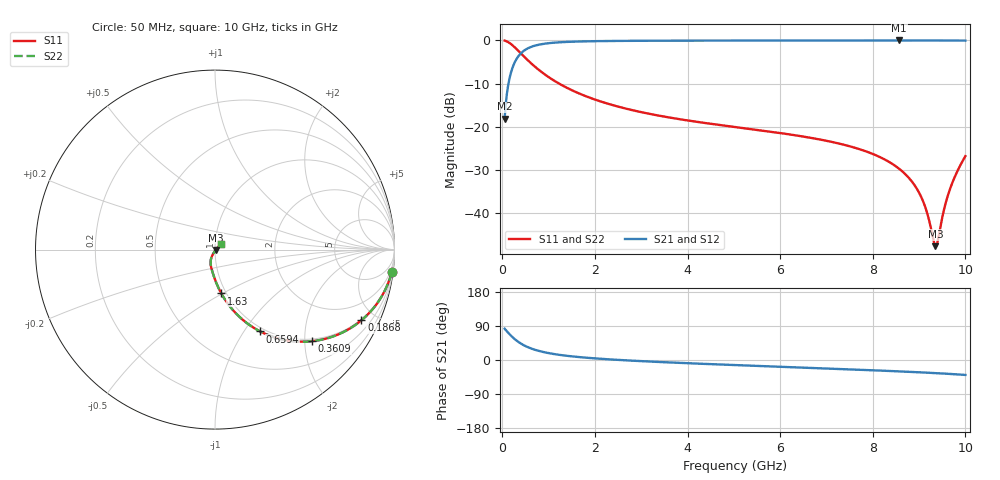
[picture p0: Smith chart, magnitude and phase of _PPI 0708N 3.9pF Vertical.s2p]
! S-Parameter data specifications (vertical orientation):
! Substrate: 40-mil Rogers 3003C, Substrate thickness, H=1.016mm, Dielectric constant, Er=3, Conductor thickness, T_mtl=0.043mm, Loss Tangent, Tand=0.003
! PCB Mounting Pad Footprint: Pad width, PadW=2.54mm , Pad length, PadL=0.51mm , Pad gap, PadG (edge-to-edge)=0.71mm , Reference planes=1.73mm apart
! Created Tue Jan 16 08:45:19 2018
# GHz S MA R 50
! 2 Port Network Data from SP1.SP block
! freq  magS11  angS11  magS21  angS21  magS12  angS12  magS22  angS22
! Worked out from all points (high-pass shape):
!   801 points, 50 MHz to 10 GHz, reference 50 ohm
!   highest |S21| = -0.03 dB at 8.57 GHz (marker M1); lowest = -18.1 dB at 50 MHz (marker M2)
!   |S21| within 3 dB of the highest: 399 MHz to end of sweep
!   lowest |S11| = -47.6 dB at 9.353 GHz (marker M3), VSWR 1.01, Z = 50.3 - j0.279 ohm
!   |S11| at or under -10 dB: 1.226 GHz to end of sweep
!   |S22| runs from -47.6 to -0.1 dB; largest |S21 - S12| = 0
!   S11 on the Smith chart (normalised r, x): 50 MHz: 1, -16; 186.8 MHz: 0.95, -4.17; 360.9 MHz: 0.95, -2.16; 659.4 MHz: 0.95, -1.19; 1.63 GHz: 0.95, -0.49; 10 GHz: 1.07, +0.07
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0.05  0.9923 -7.3  0.1241 82.7  0.1241 82.7  0.9923 -7.3
0.1370625  0.9459 -19.4  0.3241 70.5  0.3241 70.5  0.9459 -19.4
0.1868125  0.906 -25.7  0.423 64.2  0.423 64.2  0.906 -25.7
0.3609375  0.7428 -43.4  0.6691 46.6  0.6691 46.6  0.7428 -43.4
0.6594375  0.5208 -61.1  0.8531 28.8  0.8531 28.8  0.5208 -61.1
1.032563  0.366 -72.4  0.9299 17.5  0.9299 17.5  0.366 -72.4
1.629563  0.2471 -81.8  0.9681 8.0  0.9681 8.0  0.2471 -81.8
1.716625  0.2362 -82.8  0.9708 7.1  0.9708 7.1  0.2362 -82.8
3.370812  0.1352 -94.7  0.9895 -5.1  0.9895 -5.1  0.1352 -94.7
5.025  0.09969 -102.6  0.9933 -13.4  0.9933 -13.4  0.09969 -102.6
6.691625  0.07427 -109.5  0.9951 -21.0  0.9951 -21.0  0.07427 -109.5
7.674188  0.05615 -113.2  0.9958 -25.5  0.9958 -25.5  0.05615 -113.2
8.345812  0.03959 -114.9  0.9961 -28.8  0.9961 -28.8  0.03959 -114.9
8.569688  0.03284 -114.8  0.9962 -30.0  0.9962 -30.0  0.03284 -114.8
8.830875  0.02389 -113.6  0.9961 -31.4  0.9961 -31.4  0.02389 -113.6
9.029875  0.01617 -109.9  0.996 -32.6  0.996 -32.6  0.01617 -109.9
9.15425  0.01097 -103.3  0.9958 -33.3  0.9958 -33.3  0.01097 -103.3
9.35325  0.004191 -41.4  0.9955 -34.6  0.9955 -34.6  0.004191 -41.4
9.403  0.004809 -7.8  0.9953 -34.9  0.9953 -34.9  0.004809 -7.8
9.539813  0.01117 29.6  0.9949 -35.8  0.9949 -35.8  0.01117 29.6
9.664188  0.01892 37.8  0.9944 -36.7  0.9944 -36.7  0.01892 37.8
10  0.04592 42.2  0.9919 -39.4  0.9919 -39.4  0.04592 42.2
